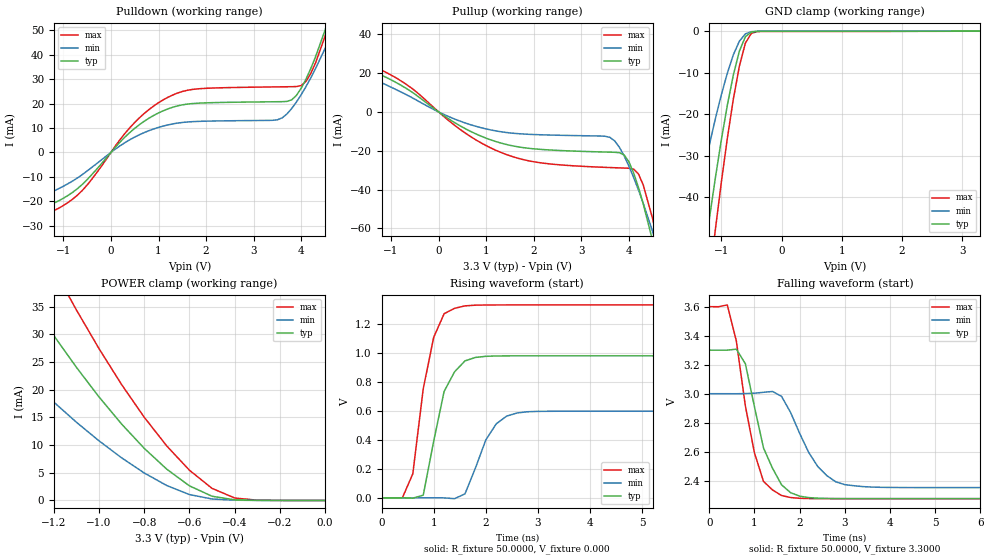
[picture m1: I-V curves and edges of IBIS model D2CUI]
| IBIS file t2i.ibs created by s2ibis2 version 1.1
| North Carolina State University Electronics Research Laboratory  1995
[IBIS ver]   2.1
[File name]   d2cui.ibs
[File Rev]   1.0
[Date]   Tuesday, March 28, 2000
[Source]   From silicon level SPICE at TOSHIBA.
[Notes]   This model does not include the values of Package Model
[Disclaimer]   None.
[Copyright]   Copyright(C) TOSHIBA Corp. 1996-2000. All Rights Reserved
|   Component TC260C
[Component]   TC260C
[Manufacturer]   TOSHIBA
[Package]
| variable   typ   min   max
R_pkg   1.00f   NA   NA
L_pkg   1.00fH   NA   NA
C_pkg   1.00fF   NA   NA
[Pin]  signal_name   model_name   R_pin   L_pin   C_pin
IO   IO   D2CUI
VDDS   VDDS   POWER
VSS   VSS   GND
| Models and submodels in the file (1): D2CUI (I/O)
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|   Model D2CUI
[Model]   D2CUI
Model_type   I/O
Polarity   Non-Inverting
Vinl   = 0.66V
Vinh   = 2.64V
C_comp   4.3pF   NA   NA
Vmeas = 1.65V
|Variable   typ   min   max
[Voltage range]  3.3   3.0   3.6
[Temperature Range]   25   100   0
[Pullup Reference]   3.3   3.0   3.6
[Pulldown Reference]   0.0   0.0   0.0
[POWER Clamp Reference]   3.3   3.0   3.6
[GND Clamp Reference]   0.0   0.0   0.0
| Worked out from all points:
|   slope of the pulldown table from 0 to 0.495 V, typ, clamps not added: 50.5 ohm
|   slope of the pullup table from 0 to 0.495 V, typ, clamps not added: 63.9 ohm
|   GND clamp passes 1 mA (typ) near -0.57 V on its own axis
|   POWER clamp passes 1 mA (typ) near -0.51 V on its own axis
|   rising waveform, R_fixture 50.0000, V_fixture 0.000: 20-80 % time 378ps typ, 437ps min, 342ps max; typ from 0 V to 0.978 V
|   falling waveform, R_fixture 50.0000, V_fixture 3.3000: 20-80 % time 534ps typ, 652ps min, 440ps max; typ from 3.3 V to 2.28 V
[Pulldown]
| voltage   I(typ)   I(min)   I(max)
-3.3V     -29.37mA   -29.01mA   -32.31mA
-1.9V     -25.53mA   -21.44mA   -28.71mA
-1V       -18.77mA   -13.85mA   -21.76mA
-500mV    -11.12mA   -7.595mA   -13.35mA
500mV     9.878mA    6.294mA    12.28mA
1.3V      18.52mA    11.69mA    23.54mA
3.5V      20.78mA    13.39mA    26.86mA
3.8V      21.56mA    18.01mA    26.94mA
4.1V      30.06mA    26.99mA    29.13mA
4.5V      50.11mA    42.6mA     47.62mA
4.7V      62.45mA    51.64mA    60.99mA
6.6V      227.2mA    181.8mA    250.9mA
[Pullup]
| voltage   I(typ)   I(min)   I(max)
-3.3V     35.88mA    43.25mA    36.87mA
-2.1V     27.55mA    25.61mA    29.91mA
-1.1V     17.77mA    13.9mA     20.3mA
600mV     -9.13mA    -6.021mA   -11.53mA
1.8V      -18.45mA   -11.4mA    -24.67mA
3.6V      -20.71mA   -13.11mA   -28.63mA
3.9V      -22.18mA   -22.69mA   -28.89mA
4.2V      -38.9mA    -40.21mA   -31.94mA
4.3V      -47.34mA   -47.03mA   -37.57mA
4.5V      -66.59mA   -61.78mA   -55.16mA
4.7V      -88.01mA   -77.77mA   -77.42mA
6.6V      -315mA     -263.4mA   -330mA
[GND_clamp]
| voltage   I(typ)   I(min)   I(max)
-3.3V     -292.9mA   -217.9mA   -337.6mA
-1.5V     -78.02mA   -49.1mA    -99.03mA
-1.3V     -55.93mA   -34.39mA   -72.82mA
-1.2V     -45.48mA   -27.6mA    -60.2mA
-1.1V     -35.57mA   -21.25mA   -48.06mA
-900mV    -17.92mA   -10.17mA   -25.93mA
-800mV    -10.62mA   -5.728mA   -16.42mA
-700mV    -4.847mA   -2.443mA   -8.473mA
-600mV    -1.357mA   -679.2uA   -2.912mA
-500mV    -225.1uA   -138.4uA   -522.2uA
-400mV    -68.02uA   -43.8uA    -112uA
3.3V      153.9pA    14.42uA    -16.89uA
[POWER_clamp]
| voltage   I(typ)   I(min)   I(max)
-3.3V     189.3mA    136.1mA    229.5mA
-1.7V     62.67mA    39.14mA    83.1mA
-1.6V     55.64mA    34.47mA    74.42mA
-1.3V     35.82mA    21.61mA    49.54mA
-1.2V     29.75mA    17.75mA    41.78mA
-1.1V     24.02mA    14.12mA    34.37mA
-900mV    13.79mA    7.692mA    20.91mA
-800mV    9.41mA     4.966mA    15.02mA
-600mV    2.644mA    1.069mA    5.459mA
-500mV    763.5uA    269.3uA    2.188mA
-400mV    115.4uA    51.5uA     450.7uA
0V        153.9pA    711.8pA    166.4pA
[Ramp]
| variable   typ   min   max
dV/dt_r   0.5871/0.3313n   0.3581/0.4089n   0.7975/0.3069n
dV/dt_f   0.6138/0.4767n   0.3881/0.6394n   0.7941/0.4120n
R_load = 50.0000
[Rising Waveform]
R_fixture = 50.0000
V_fixture = 0.000
V_fixture_min = 0.000
V_fixture_max = 0.000
| time   V(typ)   V(min)   V(max)
0s        0V         0V         0V
400ps     25.65uV    -34.07uV   -32.64uV
600ps     -2.657mV   19.97uV    165.3mV
800ps     18.2mV     107.4uV    751.5mV
1ns       389.6mV    285.4uV    1.105V
1.2ns     732.7mV    -392.7uV   1.268V
1.4ns     868.1mV    -6.149mV   1.306V
2.2ns     977.4mV    510mV      1.329V
2.6ns     978.4mV    584.5mV    1.329V
10ns      978.5mV    596.8mV    1.329V
[Falling Waveform]
R_fixture = 50.0000
V_fixture = 3.3000
V_fixture_min = 3.0000
V_fixture_max = 3.6000
| time   V(typ)   V(min)   V(max)
0s        3.3V       3V         3.6V
400ps     3.3V       3V         3.612V
600ps     3.307V     3V         3.364V
800ps     3.207V     3.001V     2.916V
1ns       2.911V     3.003V     2.594V
1.2ns     2.627V     3.01V      2.396V
1.6ns     2.372V     2.982V     2.299V
2.4ns     2.28V      2.499V     2.277V
3ns       2.277V     2.373V     2.276V
10ns      2.277V     2.353V     2.276V
